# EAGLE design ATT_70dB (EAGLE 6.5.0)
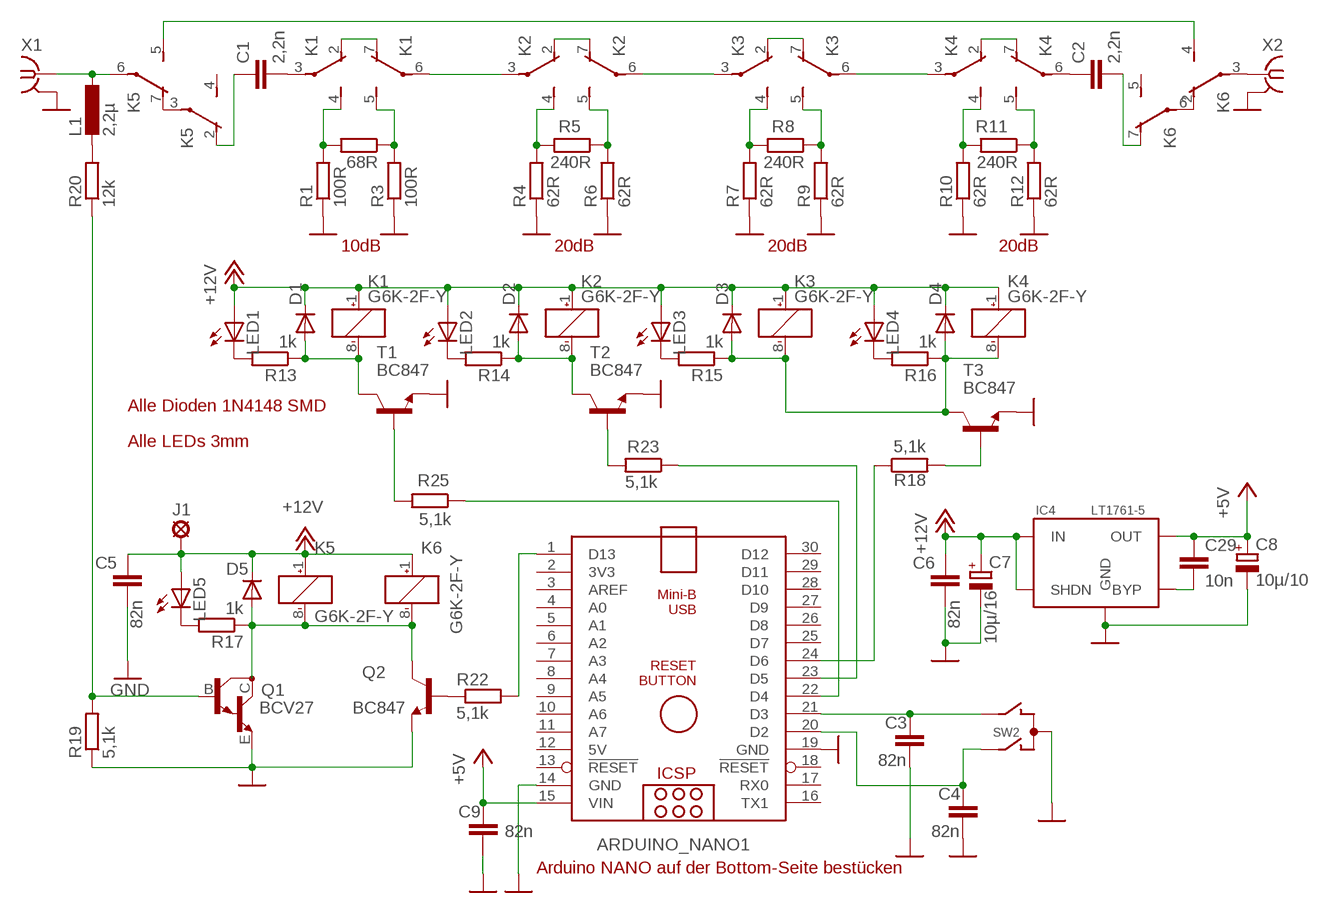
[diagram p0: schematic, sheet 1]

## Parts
ARDUINO_NANO1  ARDUINO_NANO_-DRILL  [ARDUINO_NANO_-DRILL]
C1  2,2n  C-EUC1206  [C1206]
C2  2,2n  C-EUC1206  [C1206]
C3  82n  C-EUC1206  [C1206]
C4  82n  C-EUC1206  [C1206]
C5  82n  C-EUC1206  [C1206]
C6  82n  C-EUC1206  [C1206]
C7  10µ/16  CPOL-EUCT3528  [CT3528]
C8  10µ/10  CPOL-EUCT3528  [CT3528]
C9  82n  C-EUC1206  [C1206]
C29  10n  C-EUC1206  [C1206]
D1  DIODE-MINIMELF  [MINIMELF]
D2  DIODE-MINIMELF  [MINIMELF]
D3  DIODE-MINIMELF  [MINIMELF]
D4  DIODE-MINIMELF  [MINIMELF]
D5  DIODE-MINIMELF  [MINIMELF]
IC4  LT1761-5  LT1761ES5-5  [SOT23-5]
J1  SMD-PAD-015-01  [SMD-PAD1]
K1  G6K-2F-Y  [G6K-2F-Y]
K2  G6K-2F-Y  [G6K-2F-Y]
K3  G6K-2F-Y  [G6K-2F-Y]
K4  G6K-2F-Y  [G6K-2F-Y]
K5  G6K-2F-Y  [G6K-2F-Y]
K6  G6K-2F-Y  [G6K-2F-Y]
L1  2,2µ  L-EUL3225M  [L3225M]
LED1  LED3MM  [LED3MM]
LED2  LED3MM  [LED3MM]
LED3  LED3MM  [LED3MM]
LED4  LED3MM  [LED3MM]
LED5  LED3MM  [LED3MM]
Q1  BCV27  MMBTA13LT1  [SOT23-BEC]
Q2  BC847  [SOT23]
R1  100R  R-EU_R1206  [R1206]
R2  68R  R-EU_R1206  [R1206]
R3  100R  R-EU_R1206  [R1206]
R4  62R  R-EU_R1206  [R1206]
R5  240R  R-EU_R1206  [R1206]
R6  62R  R-EU_R1206  [R1206]
R7  62R  R-EU_R1206  [R1206]
R8  240R  R-EU_R1206  [R1206]
R9  62R  R-EU_R1206  [R1206]
R10  62R  R-EU_R1206  [R1206]
R11  240R  R-EU_R1206  [R1206]
R12  62R  R-EU_R1206  [R1206]
R13  1k  R-EU_R1206  [R1206]
R14  1k  R-EU_R1206  [R1206]
R15  1k  R-EU_R1206  [R1206]
R16  1k  R-EU_R1206  [R1206]
R17  1k  R-EU_R1206  [R1206]
R18  5,1k  R-EU_R1206  [R1206]
R19  5,1k  R-EU_R1206  [R1206]
R20  12k  R-EU_R1206  [R1206]
R22  5,1k  R-EU_R1206  [R1206]
R23  5,1k  R-EU_R1206  [R1206]
R25  5,1k  R-EU_R1206  [R1206]
SW2  EC12E_SW  [ALPS_EC12E_SW]
T1  BC847  [SOT23]
T2  BC847  [SOT23]
T3  BC847  [SOT23]
X1  SMA-142-0711-821/826  [J502-ND-142-0711-821/826]
X2  SMA-142-0711-821/826  [J502-ND-142-0711-821/826]

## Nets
+5V: ARDUINO_NANO1.15(VIN) C8.+ C9.1 C29.1 IC4.5(OUT)
+12V: C5.2 C6.2 C7.+ D1.C D2.C D3.C D4.C D5.C IC4.1(IN) IC4.3(SHDN) J1.P$1(MP) K1.1(1:+) K2.1(1:+) K3.1(1:+) K4.1(1:+) K5.1(1:+) K6.1(1:+) LED1.A LED2.A LED3.A LED4.A LED5.A
GND: ARDUINO_NANO1.14(GND) ARDUINO_NANO1.19(GND) C3.2 C4.2 C5.1 C6.1 C7.- C8.- C9.2 IC4.2(GND) Q1.E Q2.2(E) R1.1 R3.1 R4.1 R6.1 R7.1 R9.1 R10.1 R12.1 R19.1 SW2.C T1.2(E) T2.2(E) T3.2(E) X1.G@1 X1.G@2 X1.G@3 X1.G@4 X2.G@1 X2.G@2 X2.G@3 X2.G@4
N$1: K1.4(2:S) R1.2 R2.2
N$2: C1.1 K5.2(2:O)
N$3: K2.4(2:S) R4.2 R5.2
N$4: K6.3(2:P) X2.1
N$5: K2.6(3:P) K3.3(2:P)
N$6: LED1.K(C) R13.2
N$7: K3.6(3:P) K4.3(2:P)
N$8: K4.5(3:S) R11.1 R12.2
N$9: K1.2(2:O) K1.7(3:O)
N$10: K2.2(2:O) K2.7(3:O)
N$11: K4.2(2:O) K4.7(3:O)
N$12: Q1.B R19.2 R20.1
N$13: D1.A K1.8(1:-) R13.1 T1.3(C)
N$14: K5.6(3:P) L1.1 X1.1
N$15: D2.A K2.8(1:-) R14.1 T2.3(C)
N$16: L1.2 R20.2
N$17: Q2.1(B) R22.1
N$18: C2.2 K6.7(3:O)
N$19: D3.A D4.A K3.8(1:-) K4.8(1:-) R15.1 R16.1 T3.3(C)
N$20: ARDUINO_NANO1.21(D3) C3.1 SW2.B
N$21: D5.A K5.8(1:-) K6.8(1:-) Q1.C Q2.3(C) R17.1
N$22: LED2.K(C) R14.2
N$23: ARDUINO_NANO1.20(D2) C4.1 SW2.A
N$24: K5.5(3:S) K6.4(2:S)
N$25: K3.2(2:O) K3.7(3:O)
N$26: LED3.K(C) R15.2
N$27: LED4.K(C) R16.2
N$28: LED5.K(C) R17.2
N$29: K5.3(2:P) K5.7(3:O)
N$30: K6.2(2:O) K6.6(3:P)
N$31: ARDUINO_NANO1.22(D4) R25.1
N$32: ARDUINO_NANO1.23(D5) R23.1
N$33: ARDUINO_NANO1.24(D6) R18.1
N$34: R25.2 T1.1(B)
N$35: R23.2 T2.1(B)
N$36: R18.2 T3.1(B)
N$37: ARDUINO_NANO1.1(D13) R22.2
N$38: C1.2 K1.3(2:P)
N$39: C29.2 IC4.4(BYP)
N$40: K1.5(3:S) R2.1 R3.2
N$41: K2.5(3:S) R5.1 R6.2
N$42: K3.4(2:S) R7.2 R8.2
N$43: K3.5(3:S) R8.1 R9.2
N$44: K4.4(2:S) R10.2 R11.2
N$45: C2.1 K4.6(3:P)
N$46: K1.6(3:P) K2.3(2:P)
Unconnected: ARDUINO_NANO1.2(3V3) ARDUINO_NANO1.3(AREF) ARDUINO_NANO1.4(A0) ARDUINO_NANO1.5(A1) ARDUINO_NANO1.6(A2) ARDUINO_NANO1.7(A3) ARDUINO_NANO1.8(A4) ARDUINO_NANO1.9(A5) ARDUINO_NANO1.10(A6) ARDUINO_NANO1.11(A7) ARDUINO_NANO1.13(!RESET) ARDUINO_NANO1.16(TX1) ARDUINO_NANO1.17(RX0) ARDUINO_NANO1.18(!RESET) ARDUINO_NANO1.25(D7) ARDUINO_NANO1.26(D8) ARDUINO_NANO1.27(D9) ARDUINO_NANO1.28(D10) ARDUINO_NANO1.29(D11) ARDUINO_NANO1.30(D12) K5.4(2:S) K6.5(3:S) SW2.D SW2.E SW2.GND1(G) SW2.GND2(G)

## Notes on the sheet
- 10dB | 20dB | 20dB | 20dB
- Alle Dioden 1N4148 SMD
- Alle LEDs 3mm
- Arduino NANO auf der Bottom-Seite bestücken

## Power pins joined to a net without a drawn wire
5V: ARDUINO_NANO1.12(5V)

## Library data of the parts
ARDUINO_NANO1 = ArduinoNanoV30:ARDUINO_NANO_-DRILL
C1-C6 C9 = rcl:C-EU: CAPACITOR, European symbol
C7 C8 = rcl:CPOL-EU: POLARIZED CAPACITOR, European symbol
C29 = rcl-2:C-EU: CAPACITOR, European symbol
D1-D5 = diode:DIODE-: DIODE
IC4 = dk3ha-2015-01:LT1761ES5-5: LT1761_X
J1 = solpad:SMD-PAD-015-01: SMD-PAD 0,15 inch x 0,1 inch
K1-K6 = relay:G6K: Low Signal Relay oeiwcsnts1.omron.com/.. D20G6K0100.pdf; MF: OMRON COMPONENTS USA; MPN: G6K-2F-Y DC3; OC_FARNELL: 1690316; OC_NEWARK: 89C6451
L1 = rcl:L-EU: INDUCTOR, European symbol
LED1-LED5 = led:LED: LED
Q1 = transistor-npn:MMBTA13*: NPN Darlington Transistor
Q2 T1-T3 = transistor:BC847: NPN TRANSISTOR
R1-R20 R22 R23 R25 = rcl:R-EU_: RESISTOR, European symbol
SW2 = switch-alps:EC12E_SW: ALPS rotary Encoder EC12E series with switch; MPN: EC12E2424407; OC_FARNELL: 1520813; OC_NEWARK: 74M1068
X1 X2 = con-coax:SMA-: SMA 50 Ohm End Launch Jack Receptacle - Round Contact; MF: JOHNSON COMPONENTS; MPN: 142-0711-821; OC_FARNELL: 1019328; OC_NEWARK: 16F3627

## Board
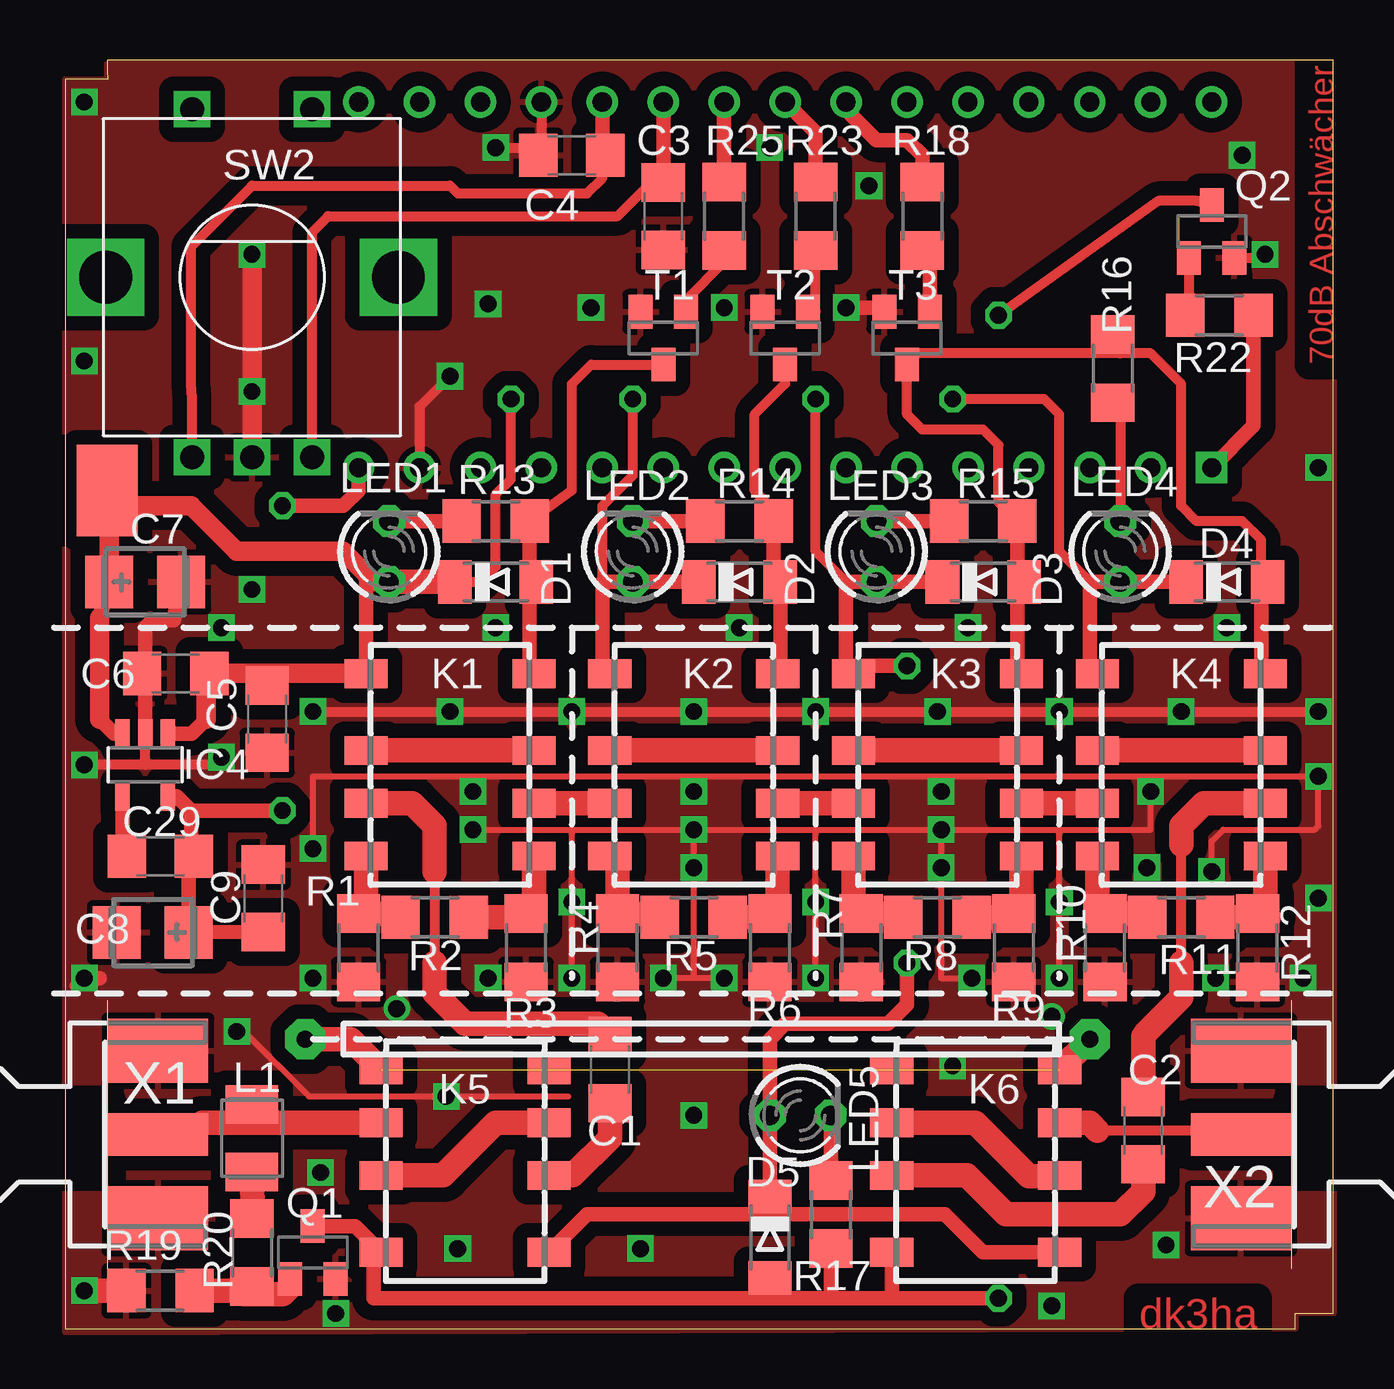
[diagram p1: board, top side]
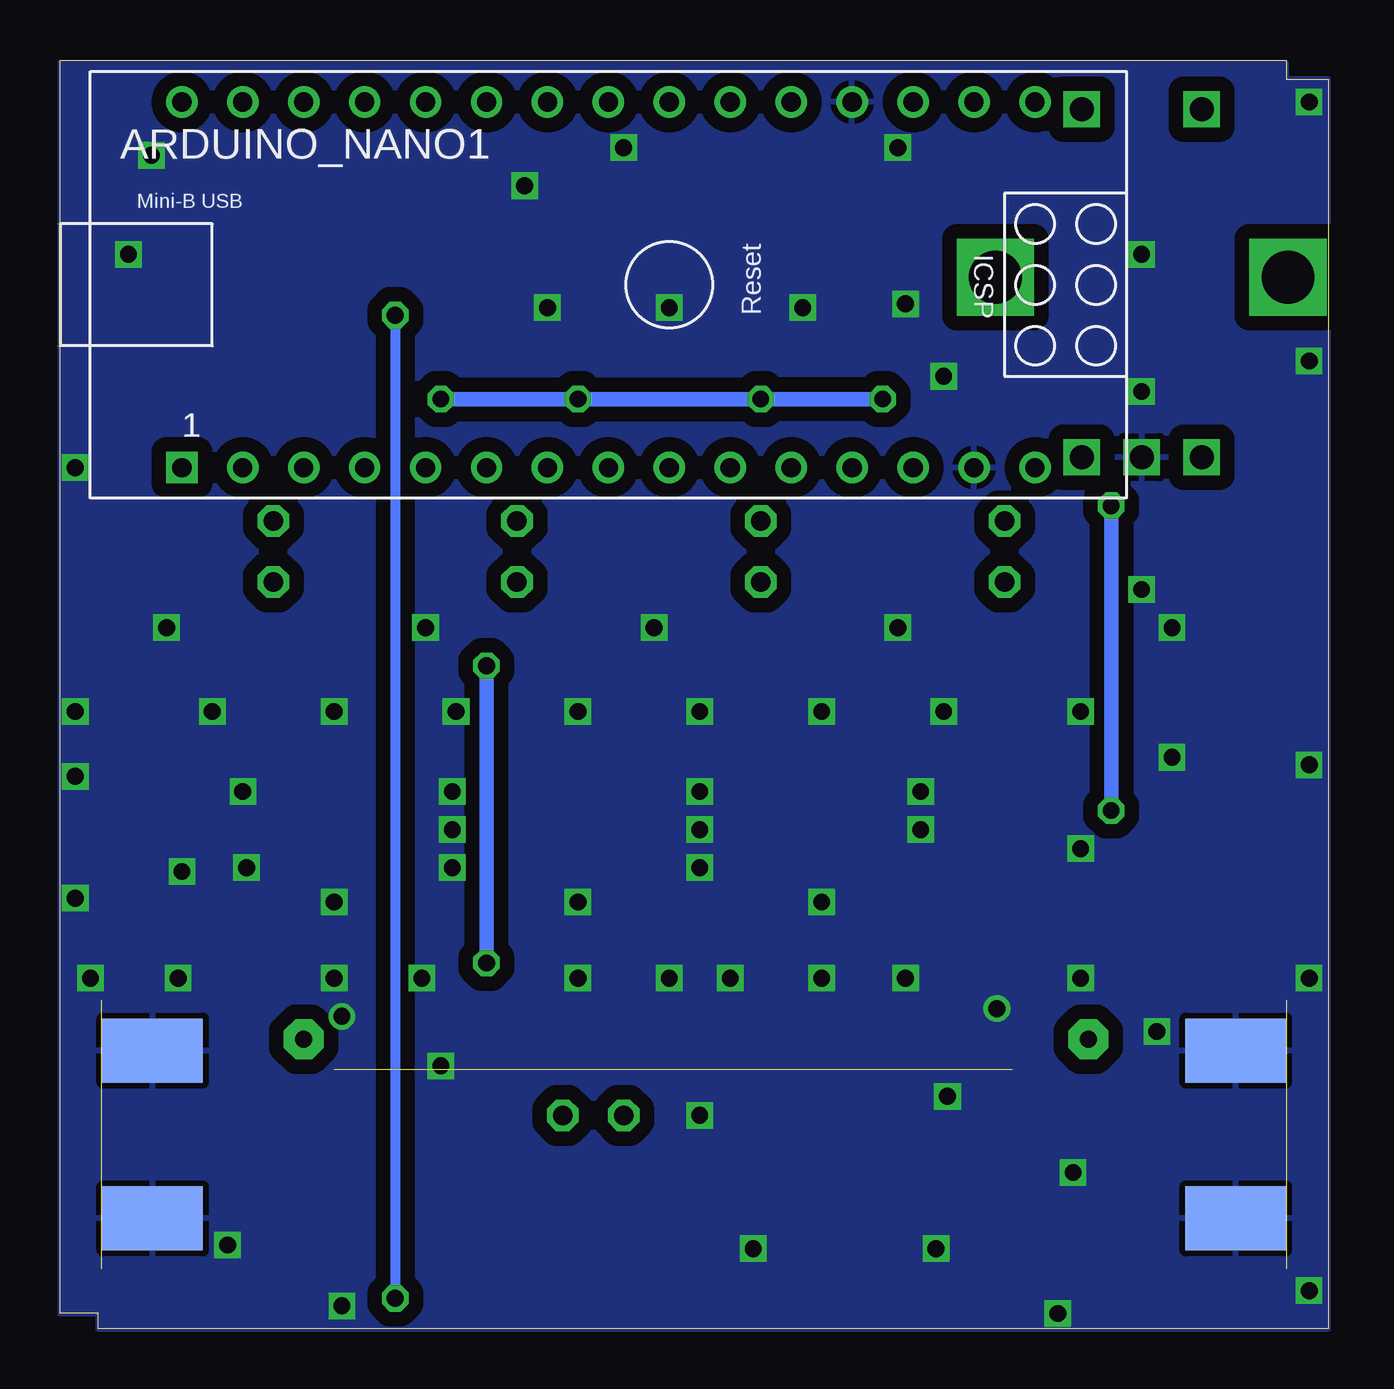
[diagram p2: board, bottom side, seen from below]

Size 52.84 x 52.86 mm. Coordinates in mm from the lower left corner, seen from the top.
Outline: 0,0 51.28,0 51.28,0.64 52.84,0.64 52.84,52.85 1.75,52.86 1.75,52.39 1.76,52.06 0,52.06 0,0
Copper layers (1*16): Top 0.035mm / dielectric 1.5mm / Bottom 0.035mm
Design rules "default *": minimum track width 10mil, minimum drill 24mil, track to track 8mil, track to pad 8mil, pad to pad 8mil, via to via 8mil, smd to smd 8mil, copper to edge 0mil, drill to drill 8mil, minimum pad ring 10mil, minimum via ring 8mil, stop-mask expansion 4mil, vias tented up to drill 0mil, thermal gap 10mil
tRestrict: area 51,6.3 to 52.9,9.5; area 0,6.3 to 1.9,9.5

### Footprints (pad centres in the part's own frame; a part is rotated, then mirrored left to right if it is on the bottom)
ARDUINO_NANO_-DRILL = drill 0.8 square: 1 -20.32,-7.62 | drill 0.8: 2 -17.78,-7.62; 3 -15.24,-7.62; 4 -12.7,-7.62; 5 -10.16,-7.62; 6 -7.62,-7.62; 7 -5.08,-7.62; 8 -2.54,-7.62; 9 0,-7.62; 10 2.54,-7.62; 11 5.08,-7.62; 12 7.62,-7.62; 13 10.16,-7.62; 14 12.7,-7.62; 15 15.24,-7.62; 16 15.24,7.62; 17 12.7,7.62; 18 10.16,7.62; 19 7.62,7.62; 20 5.08,7.62; 21 2.54,7.62; 22 0,7.62; 23 -2.54,7.62; 24 -5.08,7.62; 25 -7.62,7.62; 26 -10.16,7.62; 27 -12.7,7.62; 28 -15.24,7.62; 29 -17.78,7.62; 30 -20.32,7.62
C1206 = smd 1.6 x 1.8: 1 -1.4,0; 2 1.4,0
CT3528 = smd 2 x 2.2: + -1.5,0; - 1.5,0
MINIMELF = smd 1.4 x 1.8: A 1.7,0; C -1.7,0
SOT23-5 = smd 0.6 x 1.2: 1 -0.95,-1.306; 2 0,-1.306; 3 0.95,-1.306; 4 0.95,1.306; 5 -0.95,1.306
SMD-PAD1 = smd 3.81 x 2.54: P$1 0,0
G6K-2F-Y = smd 1.2 x 1.8: 1 -3.8,-3.5; 2 -0.6,-3.5; 3 1.6,-3.5; 4 3.8,-3.5; 5 3.8,3.5; 6 1.6,3.5; 7 -0.6,3.5; 8 -3.8,3.5
L3225M = smd 1.6 x 2.2: 1 -1.4,0; 2 1.4,0
LED3MM = drill 0.813 octagon: A -1.27,0; K 1.27,0
SOT23-BEC = smd 1 x 1.4: B -0.95,-1.1; C 0,1.1; E 0.95,-1.1
SOT23 = smd 1 x 1.4: 1 -0.95,-1.1; 2 0.95,-1.1; 3 0,1.1
R1206 = smd 1.6 x 1.803: 1 -1.422,0; 2 1.422,0
ALPS_EC12E_SW = drill 1 square: A -2.5,-7.5; B 2.5,-7.5; C 0,-7.5; D -2.5,7; E 2.5,7 | drill 2.2 square: GND1 -6.1,0; GND2 6.1,0
J502-ND-142-0711-821/826 = smd 4.191 x 1.778: 1 2.115,0 | smd 4.191 x 2.667: G@1 2.115,3.495; G@2 2.115,-3.495 | smd 4.191 x 2.667 bottom: G@3 2.115,3.495; G@4 2.115,-3.495

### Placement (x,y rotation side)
ARDUINO_NANO1  27.46,43.5 0 bottom
C1  22.7,10.79 90 top
C2  44.93,8.26 270 top
C3  24.92,46.36 270 top
C4  21.11,48.9 180 top
C5  8.41,25.4 90 top
C6  4.6,27.3 0 top
C7  3.33,31.11 0 top
C8  3.65,16.51 180 top
C9  8.25,17.94 90 top
C29  3.97,19.68 180 top
D1  17.94,31.11 0 top
D2  28.1,31.11 0 top
D3  38.26,31.11 0 top
D4  48.42,31.11 0 top
D5  29.37,3.81 270 top
IC4  3.33,23.49 180 top
J1  1.75,34.93 270 top
K1  16.03,23.49 270 top
K2  26.19,23.49 270 top
K3  36.35,23.49 270 top
K4  46.51,23.49 270 top
K5  16.67,6.99 90 top
K6  37.94,6.99 90 top
L1  7.78,7.94 270 top
LED1  13.49,32.39 90 top
LED2  23.65,32.39 90 top
LED3  33.81,32.39 90 top
LED4  43.97,32.39 90 top
LED5  30.64,8.89 0 top
Q1  10.32,3.17 0 top
Q2  47.78,45.72 0 top
R1  12.22,15.88 90 top
R2  15.4,17.14 180 top
R3  19.21,15.88 90 top
R4  23.02,15.88 90 top
R5  26.19,17.14 180 top
R6  29.37,15.88 90 top
R7  33.18,15.88 90 top
R8  36.35,17.14 180 top
R9  39.53,15.88 90 top
R10  43.34,15.88 90 top
R11  46.51,17.14 180 top
R12  49.69,15.88 90 top
R13  17.94,33.66 180 top
R14  28.1,33.66 180 top
R15  38.26,33.66 180 top
R16  43.66,40.01 270 top
R17  31.91,4.76 90 top
R18  35.72,46.36 270 top
R19  3.97,1.59 0 top
R20  7.78,3.17 90 top
R22  48.1,42.23 0 top
R23  31.27,46.36 270 top
R25  27.46,46.36 270 top
SW2  7.78,43.82 0 top
T1  24.92,41.27 180 top
T2  30,41.27 180 top
T3  35.08,41.27 180 top
X1  1.75,8.1 0 top
X2  51.12,8.1 180 top

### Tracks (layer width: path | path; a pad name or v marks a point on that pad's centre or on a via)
+5V  (via drill 0.7)
  Top 0.61: 5.24,21.59 4.64,22.19 IC4.5 4.32,22.22 | 5.24,21.59 5.24,19.81 C29.1 5.15,19.58 C8.+ C9.1 | ARDUINO_NANO1.15 12.22,34.93 11.59,34.29 v9.05,34.29 | v9.05,21.59 5.24,21.59
  Bottom 0.61: v9.05,34.29 v9.05,21.59
+12V  (via drill 0.7)
  Top 0.406: 42.7,31.11 41.43,32.39 41.43,38.1 40.8,38.73 v36.99,38.73 | 32.54,31.11 31.27,32.39 v31.27,38.73 | D1.C 17.3,31.11 17.94,31.75 17.94,34.77 18.57,35.4 v18.57,38.73 | 22.38,31.11 22.38,34.29 23.65,35.56 v23.65,38.73
  Top 0.61: K1.1 12.53,26.99 12.54,26.99 12.54,31.43 | 12.22,27.6 K1.1 | K2.1 22.38,27.6 22.38,31.11 LED2.A D2.C | K4.1 42.7,27.6 42.7,31.11 LED4.A D4.C | K6.1 38.25,3.18 36.67,4.76 29.37,4.76 | K5.1 21.75,4.76 29.37,4.76 | 29.37,4.76 D5.C LED5.A 29.37,12.06 30,12.7 34.29,12.7 35.08,13.49 v35.08,15.24 | IC4.1 5.27,24.8 5.87,25.4 | 5.87,27.17 C6.2 | K1.1 | IC4.3 2.03,24.8 1.43,25.4 | 1.43,29.61 C7.+ | D3.C LED3.A 32.54,31.11 32.54,27.3 32.55,27.29 K3.1 32.85,27.62 v35.08,27.62
  Top 0.813: C7.+ 1.83,34.7 J1.P$1 2.06,34.29 5.24,34.29 7.14,32.39 11.59,32.39 12.54,31.43 12.86,31.11 LED1.A | 5.87,25.4 5.87,27.17 | C6.2 8.41,27.3 | 8.41,27.3 K1.1 | 1.43,25.4 1.43,29.61 | C5.2 8.41,27.3
  Top 1.016: LED1.A D1.C
  Bottom 0.61: v35.08,15.24 v35.08,27.62 | v36.99,38.73 v31.27,38.73 v23.65,38.73 v18.57,38.73
GND  (via drill 0.7)
  Top 0.254: 45.24,23.02 10.32,23.02 v10.32,20 | 45.24,23.02 v52.23,23.02 52.23,20.95 52.07,20.8 48.26,20.8 47.78,20.32 v47.78,19.05 | v16.99,20.8 21.11,20.8 | 21.11,20.8 v26.19,20.8 | v26.19,20.8 31.27,20.8 | 31.27,20.8 v36.51,20.8 | v36.51,20.8 41.43,20.8 | 41.43,20.8 45.24,20.8 45.24,23.02 | v41.43,14.61 41.43,20.8 | v31.27,14.61 31.27,20.8 | v21.11,14.61 21.11,20.8 | v26.19,20.8 26.19,14.61 | 26.19,14.61 v24.92,14.61 | v27.46,14.61 26.19,14.61 | v7.14,12.38 7.46,12.38 10.16,9.68 v15.87,9.68 20.95,9.68 | v36.51,20.8 36.51,14.61 v37.78,14.61
  Top 0.406: v16.03,39.69 14.76,38.42 ARDUINO_NANO1.14 | C3.2 25.11,44.96 | Q2.2 49.86,44.62 v50.01,44.77 | 6.51,23.49 3.33,23.49 | 3.33,23.49 v0.79,23.49 | 3.33,23.49 3.33,24.76 | v10.32,25.72 v52.23,25.72 | ARDUINO_NANO1.19 19.84,49.02 C4.2 19.4,49.21 v17.94,49.21
  Top 0.61: C7.- 4.52,29.53 3.65,29.53 3.33,29.21 3.33,27.43 C6.1 3.2,26.8 3.33,26.67 IC4.2 | 1.43,14.61 0.48,14.29 v0.79,14.61 | T3.2 34.12,42.53 v32.54,42.55
  Top 0.813: 7.78,36.2 SW2.C v7.78,44.77
  Top 1.016: 49.84,14.61 R12.1 | v0.79,1.59 R19.1
  other vias: 10.32,14.61 51.59,14.61 17.62,14.61 0.79,51.12 41.12,0.95 49.05,48.9 0.79,40.32 28.1,29.21 6.51,29.21 37.62,29.21 27.46,42.55 45.88,3.49 11.27,0.64 47.94,14.61 26.19,8.89 29.37,49.21 7.78,30.8 17.94,29.21 48.42,29.21 6.51,23.81 52.23,35.88 33.5,47.62 17.62,42.7 21.11,25.72 31.27,25.72 41.43,25.72 21.91,42.55 7.78,39.05 41.12,13.02 13.81,13.34 16.99,22.38 26.19,22.38 36.51,22.38 10.64,6.51 16.35,3.33 23.97,3.33 26.19,19.21 45.24,22.38 36.51,19.21 45.09,19.21 31.27,17.78 41.43,17.78 21.11,17.78 52.23,17.94 26.19,25.72 16.03,25.72 36.35,25.72 46.51,25.72 36.99,10.95
  pour Top (isolate 0.61): 0,52.07 1.75,52.07 1.75,52.71 52.86,52.71 52.86,0.64 51.28,0.64 51.28,0 0,-0.16
  pour Bottom (isolate 0.61): 0,52.07 1.75,52.07 1.75,52.71 52.86,52.71 52.86,0.64 51.28,0.64 51.28,0 0,0
N$1
  Top 1.016: R2.2 13.49,17.3 13.19,17.3 | 13.19,17.3 R1.2 12.53,17.3 K1.4 | 13.19,17.3 R2.2 | 14.13,16.99 R2.2
N$2
  Top 1.016: K5.2 21.15,6.38 22.7,7.94 C1.1
N$3
  Top 1.016: R5.2 24.62,17.3 R4.2 23.02,19.69 K2.4
N$4
  Top 0.406: 48.89,8.26 43.02,8.26
  Top 0.61: X2.1 49,8.15 48.89,8.26
  Top 1.016: 43.02,8.26 42.7,8.57 41.45,8.57 K6.3
N$5
  Top 1.016: K2.6 K3.3
N$6
  Top 0.61: LED1.K R13.2
N$7
  Top 1.016: K3.6 K4.3
N$8
  Top 1.016: 47.78,17.3 R11.1 50.17,17.14 R12.2 50.01,17.3 K4.5
N$9
  Top 1.016: K1.2 K1.7
N$10
  Top 1.016: K2.7 K2.2
N$11
  Top 1.016: K4.2 K4.7
N$12
  Top 1.016: R19.2 6.98,1.59 R20.1 7.46,1.44 9.06,1.44 9.37,1.75 Q1.B
N$13
  Top 0.406: R13.1 21.11,34.93 21.11,39.37 21.92,40.18 T1.3
  Top 0.61: R13.1 19.36,31.11 | 19.36,31.11 19.36,27.3 19.99,27.29 K1.8 | D1.A 19.36,31.11
N$14
  Top 1.016: X1.1 5.24,8.1 5.71,8.57 7.3,8.57 | 7.3,8.57 13.17,8.57 K5.6 | L1.1 7.3,8.57
N$15
  Top 0.406: R14.1 30,33.66 28.73,34.93 28.73,38.1 30,39.37 T2.3
  Top 0.61: R14.1 29.52,31.39 D2.A 29.8,28.04 K2.8
N$16
  Top 1.016: R20.2 7.81,4.6 L1.2
N$17
  Top 0.406: Q2.1 46.83,42.38 R22.1
N$18
  Top 1.016: K6.7 37.59,6.38 39.21,4.76 43.97,4.76 44.93,5.71 C2.2
N$19
  Top 0.406: D4.A 49.84,31.11 49.84,32.87 49.05,33.66 47.15,33.66 46.51,34.29 46.51,39.37 45.24,40.64 43.97,40.64 | 43.97,40.64 35.08,40.64 T3.3 35.08,38.1 35.72,37.47 38.26,37.47 38.89,36.83 38.89,34.44 R15.1 | R16.1 43.66,40.96 43.97,40.64
  Top 0.61: 39.68,30.8 R15.1 39.53,33.81 | 39.68,30.8 39.68,27.76 K3.8 | D3.A 39.96,31.07 39.68,30.8 | 49.84,31.11 49.84,27.47
  Top 1.016: 49.84,27.47 K4.8
N$20
  Top 0.406: SW2.B 10.28,45.68 10.95,46.36 23.02,46.36 24.29,47.62 24.79,47.62 C3.1
  Top 0.61: ARDUINO_NANO1.21 C3.1
N$21  (via drill 0.7)
  Top 0.406: Q2.3 47.15,46.99 45.56,46.99 v38.89,42.23
  Top 0.61: R17.1 31.91,1.27 | 12.86,3.18 12.86,1.27 29.37,1.27 | 31.91,1.27 34.45,1.27 | 34.45,1.27 v38.89,1.27 | K6.8 34.45,1.27 | 29.37,1.27 31.91,1.27 | Q1.C 12.08,4.28 K5.8 | D5.A 29.37,1.27
  Top 1.016: K5.8 12.86,3.18
  Bottom 0.406: v38.89,42.23 v38.89,1.27
N$22
  Top 0.61: LED2.K R14.2
N$23
  Top 0.406: SW2.A 5.28,38.77 5.24,39.37 5.24,45.09 7.78,47.62 16.03,47.62 16.35,47.31 21.75,47.31 22.38,47.94 22.38,48.77 C4.1
  Top 0.61: ARDUINO_NANO1.20 22.38,49.02 C4.1
N$24  (via drill 0.7 pad 1.68)  (1 unrouted)
  Top 1.016: v42.7,12.06 42.7,12.05 K6.4 | v10,12.06 11.89,12.06 K5.5
N$25
  Top 1.016: K3.2 K3.7
N$26
  Top 0.61: LED3.K R15.2
N$27
  Top 0.406: R16.2 43.97,38.58 LED4.K
N$28
  Top 0.61: R17.2 LED5.K
N$29
  Top 1.016: K5.7 15.75,6.38 17.94,8.57 18.25,8.57 K5.3
N$30
  Top 1.016: K6.6 37.93,8.59 40.16,6.35 41.41,6.35 K6.2
N$31
  Top 0.61: ARDUINO_NANO1.22 R25.1 27.46,47.62
N$32
  Top 0.61: ARDUINO_NANO1.23 31.27,49.85 R23.1
N$33
  Top 0.61: ARDUINO_NANO1.24 32.54,50.8 33.81,49.53 35.08,49.53 35.72,48.9 R18.1
N$34
  Top 0.406: T1.1 25.86,42.85 27.46,44.45 R25.2
N$35
  Top 0.406: T2.1 31.27,42.38 R23.2
N$36
  Top 0.61: T3.1 36.03,44.62 R18.2
N$37
  Top 0.61: R22.2 49.52,37.63 ARDUINO_NANO1.1
N$38
  Top 0.406: 15.4,19.05 15.4,15.24
  Top 1.016: 12.52,21.91 K1.3 14.46,21.89 15.4,20.95 15.4,19.05 | 15.4,15.24 15.4,13.97 16.67,12.7 22.2,12.7 C1.2
N$39
  Top 0.61: IC4.4 2.38,19.87 C29.2
N$40
  Top 1.016: K1.5 19.53,17.3 R3.2 19.21,17.14 R2.1
N$41
  Top 1.016: K2.5 29.69,17.3 R6.2 29.37,17.14 R5.1
N$42
  Top 1.016: R8.2 34.78,17.3 R7.2 32.85,17.3 K3.4
N$43
  Top 1.016: R8.1 39.53,17.14 R9.2 39.85,17.3 K3.5
N$44
  Top 1.016: R11.2 44.94,17.3 R10.2 43.01,17.3 K4.4
N$45
  Top 0.406: 46.51,15.24 46.51,20.16
  Top 1.016: C2.1 44.93,12.2 45.08,12.38 46.51,13.81 46.51,15.24 | 46.51,20.16 46.51,20.95 47.45,21.89 K4.6
N$46
  Top 1.016: K1.6 K2.3

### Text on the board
Top: 70dB Abschwächer | dk3ha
